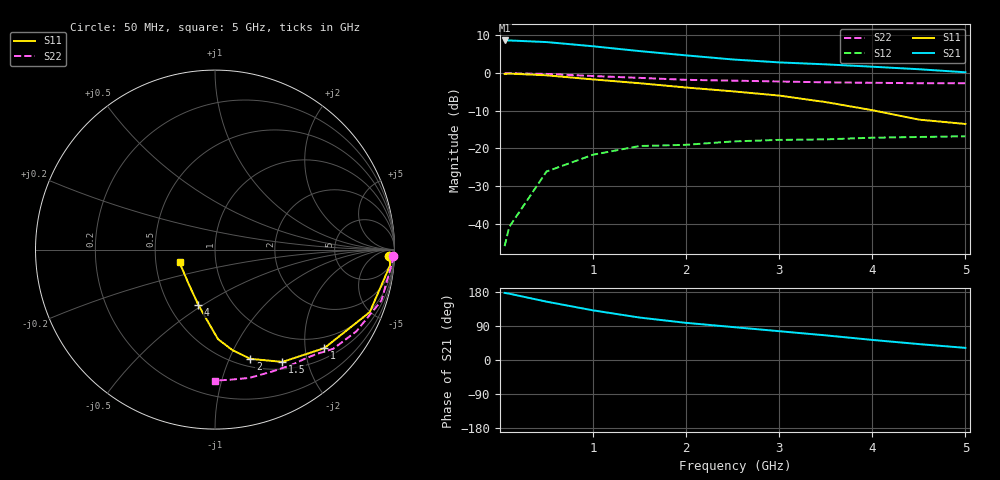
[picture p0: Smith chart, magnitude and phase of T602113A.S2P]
!AT-60211
!S-PARAMETERS at Vce=3V  Ic=0.8mA.  LAST UPDATED 07-21-92
# ghz s ma r 50
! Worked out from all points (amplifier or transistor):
!   12 points, 50 MHz to 5 GHz, reference 50 ohm
!   highest |S21| = 8.6 dB at 50 MHz (marker M1)
!   |S21| within 3 dB of that: start of sweep to 1.576 GHz
!   unconditionally stable (mu >= 1): 2.854 GHz to end of sweep
!   at 500 MHz: K = 0.20, MSG = 17.2 dB, |S12| = -26.2 dB
!   at 2.5 GHz: K = 0.90, MSG = 10.9 dB, |S12| = -18.2 dB
!   at 5 GHz: K = 1.49, MAG = 4.4 dB, |S12| = -16.8 dB
!   S11 on the Smith chart (normalised r, x): 50 MHz: 28, -33; 1 GHz: 0.72, -2.42; 1.5 GHz: 0.60, -1.60; 2 GHz: 0.58, -1.20; 4 GHz: 0.70, -0.47; 5 GHz: 0.66, -0.10
0.05  0.97 -2.0  2.7 177.0  0.005 94.0  0.99 -2.0
0.1  0.98 -5.0  2.7 175.0  0.009 93.0  0.99 -4.0
0.5  0.93 -22.0  2.57 154.0  0.049 70.0  0.97 -17.0
1  0.82 -42.0  2.26 131.0  0.082 57.0  0.91 -30.0
1.5  0.73 -59.0  1.95 112.0  0.107 46.0  0.86 -40.0
2  0.64 -72.0  1.71 98.0  0.111 38.0  0.81 -46.0
2.5  0.57 -80.0  1.51 87.0  0.123 37.0  0.79 -50.0
3  0.5 -88.0  1.38 76.0  0.129 34.0  0.77 -57.0
3.5  0.41 -95.0  1.3 65.0  0.131 34.0  0.75 -65.0
4  0.32 -107.0  1.21 53.0  0.138 31.0  0.74 -75.0
4.5  0.24 -128.0  1.12 42.0  0.141 30.0  0.73 -83.0
5  0.21 -160.0  1.02 32.0  0.144 31.0  0.73 -90.0
